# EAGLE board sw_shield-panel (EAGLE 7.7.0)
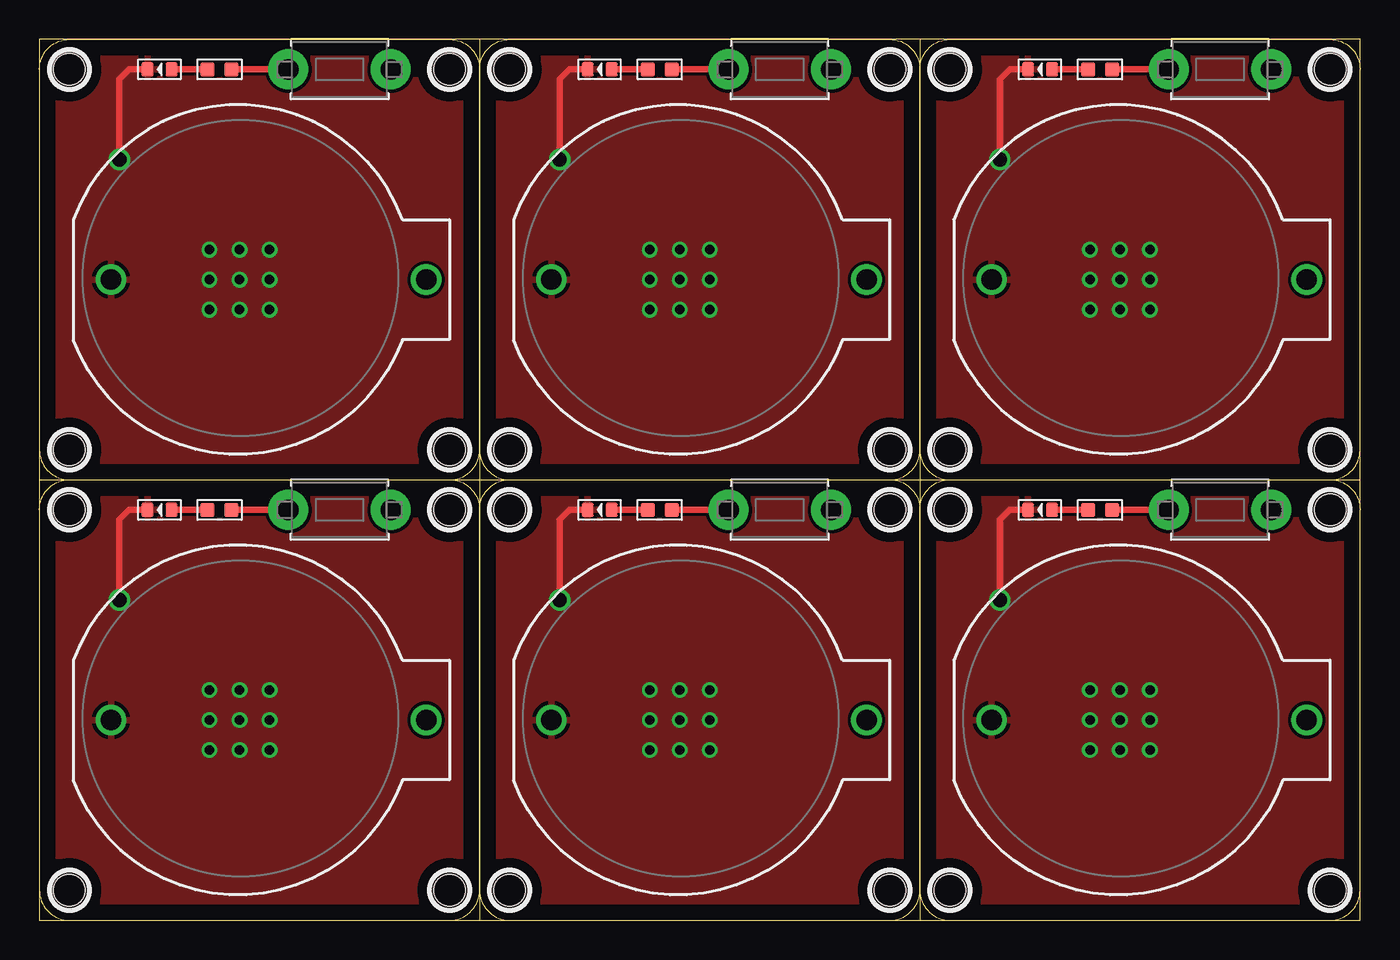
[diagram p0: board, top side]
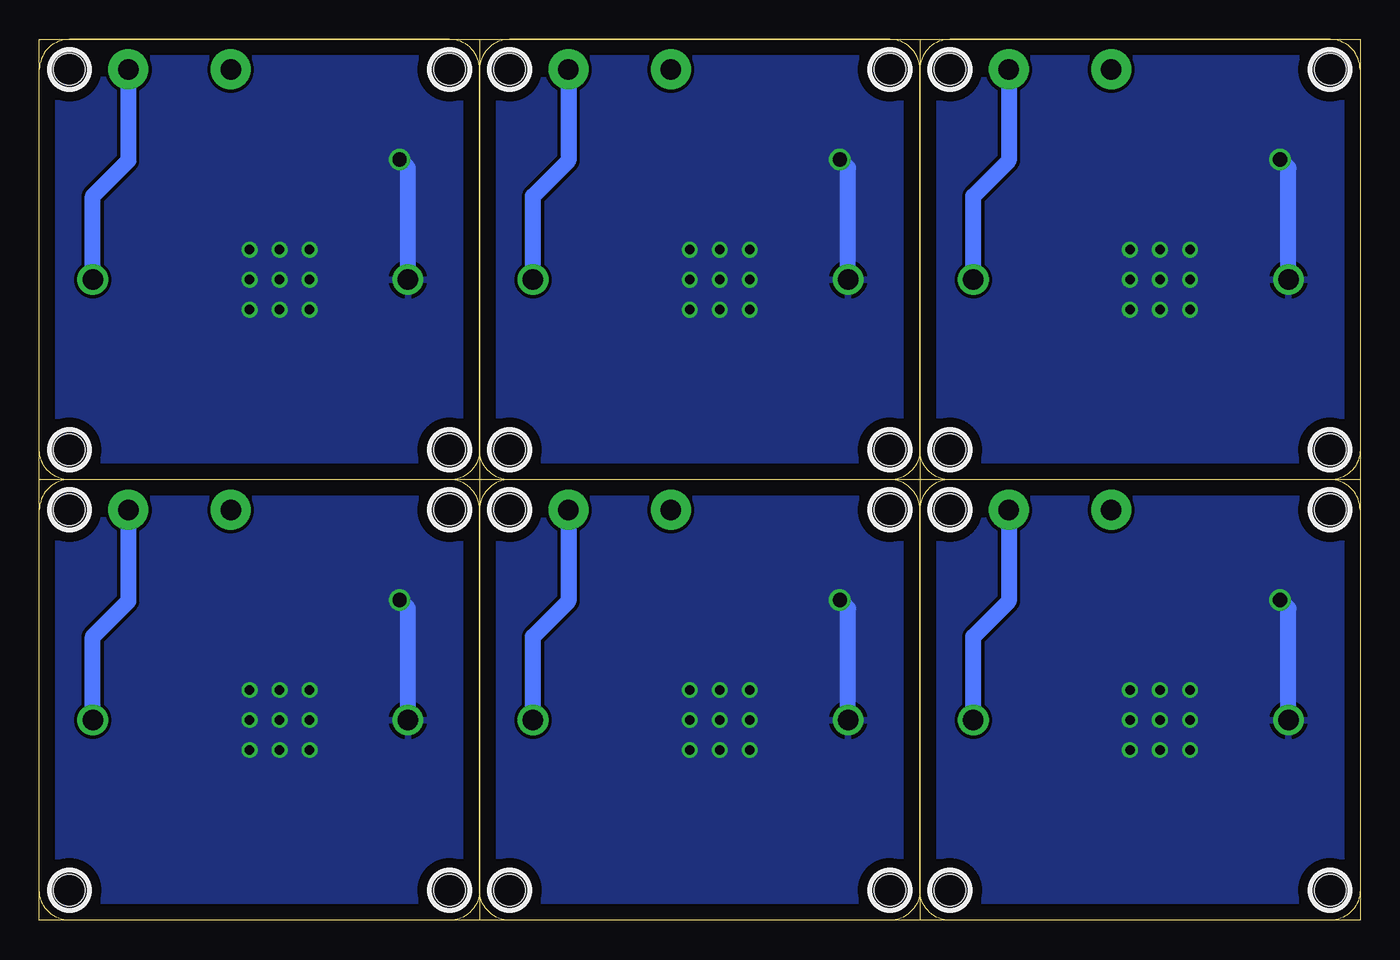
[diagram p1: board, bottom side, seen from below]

Size 83.82 x 55.88 mm. Coordinates in mm from the lower left corner, seen from the top.
Outline: 48 segments
Copper layers (1*16): Top 0.035mm / dielectric 1.5mm / Bottom 0.035mm
Design rules "default": minimum track width 10mil, minimum drill 24mil, track to track 8mil, track to pad 8mil, pad to pad 8mil, via to via 8mil, smd to smd 8mil, copper to edge 40mil, drill to drill 8mil, minimum pad ring 10mil, minimum via ring 8mil, stop-mask expansion 4mil, vias tented up to drill 0mil, thermal gap 10mil
Holes 2 mm at 1.91,1.91 26.04,1.91 26.04,26.04 1.91,26.04 29.84,1.91 53.98,1.91 53.98,26.04 29.84,26.04 57.78,1.91 81.92,1.91 81.92,26.04 57.78,26.04 1.91,29.84 26.04,29.84 26.04,53.98 1.91,53.98 29.84,29.84 53.98,29.84 53.98,53.98 29.84,53.98 57.78,29.84 81.92,29.84 81.92,53.98 57.78,53.98
Milling: 13 lines

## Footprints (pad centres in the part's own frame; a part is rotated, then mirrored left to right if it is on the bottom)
BATTCOM_20MM_PTH = drill 1.3: 1 11.85,0; 2 -8.15,0
LED-0603 = smd 0.762 x 0.889: + -0.762,0; - 0.762,0
R0603 = smd 0.889 x 0.889: 1 0,0.762; 2 0,-0.762
TACT_PANA-EVQ = drill 1.3 pad 2.54: P$1 -3.25,0; P$2 3.25,0

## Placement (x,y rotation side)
BT1  [BATTCOM_20MM_PTH]  12.7,12.7 0 top
BT2  [BATTCOM_20MM_PTH]  40.64,12.7 0 top
BT3  [BATTCOM_20MM_PTH]  68.58,12.7 0 top
BT4  [BATTCOM_20MM_PTH]  12.7,40.64 0 top
BT5  [BATTCOM_20MM_PTH]  40.64,40.64 0 top
BT6  [BATTCOM_20MM_PTH]  68.58,40.64 0 top
D1  BLUE-0603  [LED-0603]  7.62,26.04 180 top
D2  BLUE-0603  [LED-0603]  35.56,26.04 180 top
D3  BLUE-0603  [LED-0603]  63.5,26.04 180 top
D4  BLUE-0603  [LED-0603]  7.62,53.98 180 top
D5  BLUE-0603  [LED-0603]  35.56,53.98 180 top
D6  BLUE-0603  [LED-0603]  63.5,53.98 180 top
R1  330R  [R0603]  11.43,26.04 270 top
R2  330R  [R0603]  39.37,26.04 270 top
R3  330R  [R0603]  67.31,26.04 270 top
R4  330R  [R0603]  11.43,53.98 270 top
R5  330R  [R0603]  39.37,53.98 270 top
R6  330R  [R0603]  67.31,53.98 270 top
SW1  [TACT_PANA-EVQ]  19.05,26.04 180 top
SW2  [TACT_PANA-EVQ]  46.99,26.04 180 top
SW3  [TACT_PANA-EVQ]  74.93,26.04 180 top
SW4  [TACT_PANA-EVQ]  19.05,53.98 180 top
SW5  [TACT_PANA-EVQ]  46.99,53.98 180 top
SW6  [TACT_PANA-EVQ]  74.93,53.98 180 top

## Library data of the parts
BT1-BT6 = SparkFun-Batteries; PROD_ID: BATT-09031; SF_SKU: PRT-00783
D1-D6 = Seeed-LED; MPN: 19-217-BHC-ZL1M2RY-3T
R1-R6 = Seeed-Resistor; MPN: RC0603FR-07330RL
SW1-SW6 = adafruit

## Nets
GND: BT1.2 D1.-
GND1: BT2.2 D2.-
GND2: BT3.2 D3.-
GND3: BT4.2 D4.-
GND4: BT5.2 D5.-
GND5: BT6.2 D6.-
N$1: D2.+ R2.2
N$2: D1.+ R1.2
N$3: R1.1 SW1.P$2
N$4: BT1.1 SW1.P$1
N$5: R2.1 SW2.P$2
N$6: BT2.1 SW2.P$1
N$7: D3.+ R3.2
N$8: R3.1 SW3.P$2
N$9: BT3.1 SW3.P$1
N$10: D4.+ R4.2
N$11: R4.1 SW4.P$2
N$12: BT4.1 SW4.P$1
N$13: D5.+ R5.2
N$14: R5.1 SW5.P$2
N$15: BT5.1 SW5.P$1
N$16: D6.+ R6.2
N$17: R6.1 SW6.P$2
N$18: BT6.1 SW6.P$1

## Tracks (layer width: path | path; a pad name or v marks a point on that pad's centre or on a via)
GND  (via drill 0.6, 0.9)
  Top 0.406: v5.08,20.32 5.08,25.4 5.71,26.04 D1.-
  Bottom 1.016: BT1.2 4.55,19.79 v5.08,20.32
  other vias: 12.7,12.7 12.7,14.61 10.79,14.61 10.79,12.7 14.61,14.61 14.61,12.7 14.61,10.79 12.7,10.79 10.79,10.79
  pour Top: 0,0 27.94,0 27.94,27.94 0,27.94
  pour Bottom: 0,0 27.94,0 27.94,27.94 0,27.94
GND1  (via drill 0.6, 0.9)
  Top 0.406: v33.02,20.32 33.02,25.4 33.66,26.04 D2.-
  Bottom 1.016: BT2.2 32.49,19.79 v33.02,20.32
  other vias: 40.64,12.7 40.64,14.61 38.73,14.61 38.73,12.7 42.55,14.61 42.55,12.7 42.55,10.79 40.64,10.79 38.73,10.79
  pour Top: 27.94,0 55.88,0 55.88,27.94 27.94,27.94
  pour Bottom: 27.94,0 55.88,0 55.88,27.94 27.94,27.94
GND2  (via drill 0.6, 0.9)
  Top 0.406: v60.96,20.32 60.96,25.4 61.59,26.04 D3.-
  Bottom 1.016: BT3.2 60.43,19.79 v60.96,20.32
  other vias: 68.58,12.7 68.58,14.61 66.67,14.61 66.67,12.7 70.48,14.61 70.48,12.7 70.48,10.79 68.58,10.79 66.67,10.79
  pour Top: 55.88,0 83.82,0 83.82,27.94 55.88,27.94
  pour Bottom: 55.88,0 83.82,0 83.82,27.94 55.88,27.94
GND3  (via drill 0.6, 0.9)
  Top 0.406: v5.08,48.26 5.08,53.34 5.71,53.98 D4.-
  Bottom 1.016: BT4.2 4.55,47.73 v5.08,48.26
  other vias: 12.7,40.64 12.7,42.55 10.79,42.55 10.79,40.64 14.61,42.55 14.61,40.64 14.61,38.73 12.7,38.73 10.79,38.73
  pour Top: 0,27.94 27.94,27.94 27.94,55.88 0,55.88
  pour Bottom: 0,27.94 27.94,27.94 27.94,55.88 0,55.88
GND4  (via drill 0.6, 0.9)
  Top 0.406: v33.02,48.26 33.02,53.34 33.66,53.98 D5.-
  Bottom 1.016: BT5.2 32.49,47.73 v33.02,48.26
  other vias: 40.64,40.64 40.64,42.55 38.73,42.55 38.73,40.64 42.55,42.55 42.55,40.64 42.55,38.73 40.64,38.73 38.73,38.73
  pour Top: 27.94,27.94 55.88,27.94 55.88,55.88 27.94,55.88
  pour Bottom: 27.94,27.94 55.88,27.94 55.88,55.88 27.94,55.88
GND5  (via drill 0.6, 0.9)
  Top 0.406: v60.96,48.26 60.96,53.34 61.59,53.98 D6.-
  Bottom 1.016: BT6.2 60.43,47.73 v60.96,48.26
  other vias: 68.58,40.64 68.58,42.55 66.67,42.55 66.67,40.64 70.48,42.55 70.48,40.64 70.48,38.73 68.58,38.73 66.67,38.73
  pour Top: 55.88,27.94 83.82,27.94 83.82,55.88 55.88,55.88
  pour Bottom: 55.88,27.94 83.82,27.94 83.82,55.88 55.88,55.88
N$1
  Top 0.406: R2.2 D2.+
N$2
  Top 0.406: R1.2 D1.+
N$3
  Top 0.406: SW1.P$2 R1.1
N$4
  Bottom 1.016: BT1.1 24.55,18 22.3,20.25 SW1.P$1
N$5
  Top 0.406: SW2.P$2 R2.1
N$6
  Bottom 1.016: BT2.1 52.49,18 50.24,20.25 SW2.P$1
N$7
  Top 0.406: R3.2 D3.+
N$8
  Top 0.406: SW3.P$2 R3.1
N$9
  Bottom 1.016: BT3.1 80.43,18 78.18,20.25 SW3.P$1
N$10
  Top 0.406: R4.2 D4.+
N$11
  Top 0.406: SW4.P$2 R4.1
N$12
  Bottom 1.016: BT4.1 24.55,45.94 22.3,48.19 SW4.P$1
N$13
  Top 0.406: R5.2 D5.+
N$14
  Top 0.406: SW5.P$2 R5.1
N$15
  Bottom 1.016: BT5.1 52.49,45.94 50.24,48.19 SW5.P$1
N$16
  Top 0.406: R6.2 D6.+
N$17
  Top 0.406: SW6.P$2 R6.1
N$18
  Bottom 1.016: BT6.1 80.43,45.94 78.18,48.19 SW6.P$1

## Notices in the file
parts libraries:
SparkFun-Batteries: Licensing: Creative Commons ShareAlike 4.0 International - https://creativecommons.org/licenses/by-sa/4.0
